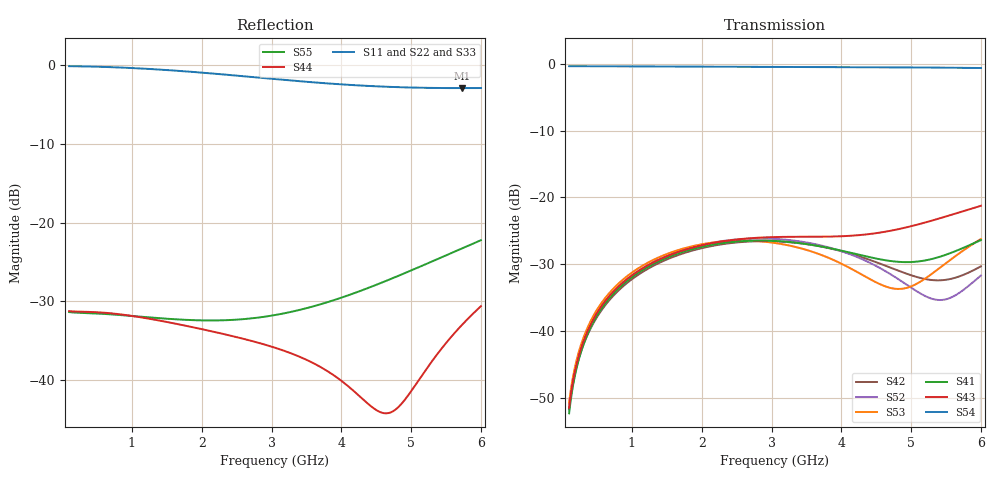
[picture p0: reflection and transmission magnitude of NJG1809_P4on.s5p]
! Port1:P1  Port2:P2  Port3:P3  Port4:P4  Port5:PC
# hz S ma R 50
! 5 Port Network Data from SP1.SP block
! freq  magS11  angS11  magS12  angS12  magS13  angS13  magS14  angS14
!  magS15  angS15
!  magS21  angS21  magS22  angS22  magS23  angS23
!  magS24  angS24  magS25  angS25
!  magS31  angS31  magS32  angS32
!  magS33  angS33  magS34  angS34  magS35  angS35
!  magS41  angS41
!  magS42  angS42  magS43  angS43  magS44  angS44  magS45  angS45
!  magS51  angS51  magS52  angS52  magS53  angS53  magS54  angS54
!  magS55  angS55
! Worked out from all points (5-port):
!   591 points, 100 MHz to 6 GHz, reference 50 ohm
!   strongest paths, dB at 100 MHz, 1.57 GHz, 3.05 GHz, 4.53 GHz, 6 GHz:
!     S54: -0.4, -0.4, -0.5, -0.5, -0.6
!     S43: -51.5, -28.5, -25.9, -25.3, -21.3
!     S41: -52.3, -28.7, -26.5, -29.2, -26.4
!     S53: -50.7, -28.2, -26.8, -32.9, -26.2
!     S52: -51.3, -28.5, -26.2, -30.4, -31.7
!     S42: -51.8, -29.0, -26.6, -29.8, -30.3
!   lowest |S11| = -3.0 dB at 5.73 GHz (marker M1), VSWR 5.92, Z = 10.8 + j26 ohm
!   |S11| at or under -10 dB: nowhere
